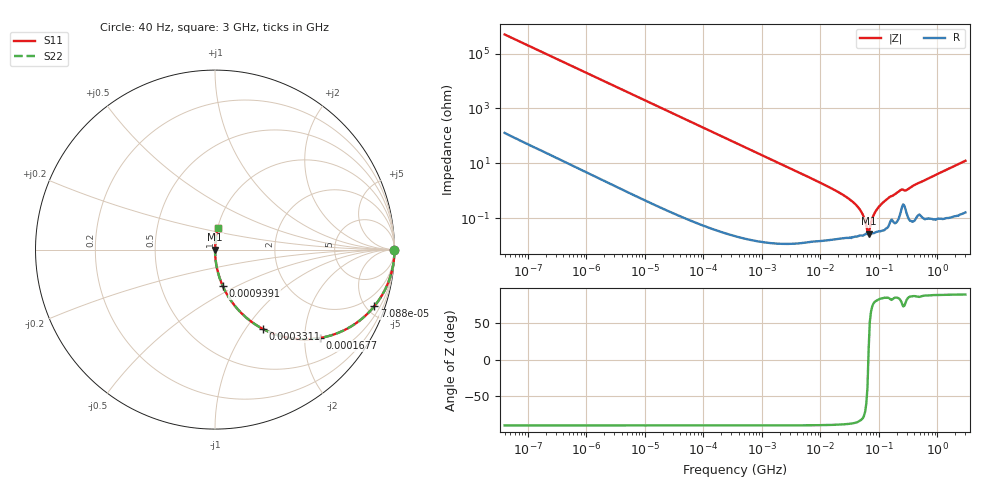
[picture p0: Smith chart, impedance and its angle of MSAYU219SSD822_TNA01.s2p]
! MSAYU219SSD822_TNA01  S-PARAMETER MODEL  ( General Type )
! Model Generated by TAIYO YUDEN Corporation (http://www.ty-top.com)
! Version 2.0
! TAIYO YUDEN Control No. 031016
! Copyright(c) 2003 TAIYO YUDEN CO.,LTD. All Rights Reserved.
! Product Description (link to TY-COMPAS)
! https://ds.yuden.co.jp/TYCOMPAS/or/detail?pn=MSAYU219SSD822KTNA01&u=M
! Products Name : Multilayer Ceramic Capacitors
! Characteristics :
!  Capacitance : 8200 pF , Rated Voltage : 50V
!  Case Size : 2.0 x 1.25 / 0.079 x 0.049 [mm/inch] , Thickness : 0.85 / 0.033 [mm/inch]
!  (Conditions: Temperature = 25 degC , DC Bias Current/Voltage = 0A / 0V)
! External Node Assignments :
!  1  o---| |---o  2
! GND o---------o GND
! Frequency Range : 40Hz  -  3GHz  [ 401 STEP ]
# MHz S RI R 50
! Freq[MHz].  S11 Real  S11 Imag  S21 Real  S21 Imag  S12 Real  S12 Imag  S22 Real  S22 Imag
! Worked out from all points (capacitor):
!   401 points, 40 Hz to 3 GHz, reference 50 ohm
!   read as one part in series: C = 7.97 nF near 44 Hz
!   lowest |Z| = 27.1 mohm at 66.58 MHz (marker M1)
!   series resonance near 65.89 MHz, so ESL is about 730 pH
!   S11 on the Smith chart (normalised r, x): 40 Hz: open; 70.88 kHz: 1.00, -5.63; 167.7 kHz: 1.00, -2.38; 331.1 kHz: 1.00, -1.21; 939.1 kHz: 1.00, -0.43; 3 GHz: 1.00, +0.25
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4e-05  1 -0.0002  9.2e-08 0.0002  9.2e-08 0.0002  1 -0.0002
0.000834  1 -0.00418  1.84e-05 0.00418  1.84e-05 0.00418  1 -0.00418
0.017386  0.9925 -0.0864  0.00754 0.0864  0.00754 0.0864  0.9925 -0.0864
0.07088  0.888 -0.3152  0.112 0.3152  0.112 0.3152  0.888 -0.3152
0.167721  0.5863 -0.4924  0.4137 0.4924  0.4137 0.4924  0.5863 -0.4924
0.331057  0.2668 -0.4421  0.7332 0.4421  0.7332 0.4421  0.2668 -0.4421
0.362475  0.2329 -0.4225  0.7671 0.4225  0.7671 0.4225  0.2329 -0.4225
0.939115  0.0433 -0.2033  0.9567 0.2033  0.9567 0.2033  0.0433 -0.2033
7.222098  0.000885 -0.0273  0.9991 0.0273  0.9991 0.0273  0.000885 -0.0273
21.43715  0.00025 -0.00831  0.9998 0.00831  0.9998 0.00831  0.00025 -0.00831
36.93337  0.000218 -0.00369  0.9998 0.00369  0.9998 0.00369  0.000218 -0.00369
48.47801  0.000237 -0.00187  0.9998 0.00187  0.9998 0.00187  0.000237 -0.00187
55.54024  0.000246 -0.00103  0.9998 0.00103  0.9998 0.00103  0.000246 -0.00103
60.81113  0.000274 -0.000469  0.9997 0.000469  0.9997 0.000469  0.000274 -0.000469
66.58224  0.000263 6.3e-05  0.9997 -6.3e-05  0.9997 -6.3e-05  0.000263 6.3e-05
69.67004  0.000271 0.000339  0.9997 -0.000339  0.9997 -0.000339  0.000271 0.000339
79.8195  0.000283 0.00117  0.9997 -0.00117  0.9997 -0.00117  0.000283 0.00117
91.44753  0.000322 0.00201  0.9997 -0.00201  0.9997 -0.00201  0.000322 0.00201
150.5692  0.000633 0.00574  0.9994 -0.00574  0.9994 -0.00574  0.000633 0.00574
226.4253  0.00134 0.00992  0.9987 -0.00992  0.9987 -0.00992  0.00134 0.00992
297.2015  0.0016 0.0105  0.9984 -0.0105  0.9984 -0.0105  0.0016 0.0105
3000  0.0166 0.1213  0.9834 -0.1213  0.9834 -0.1213  0.0166 0.1213
